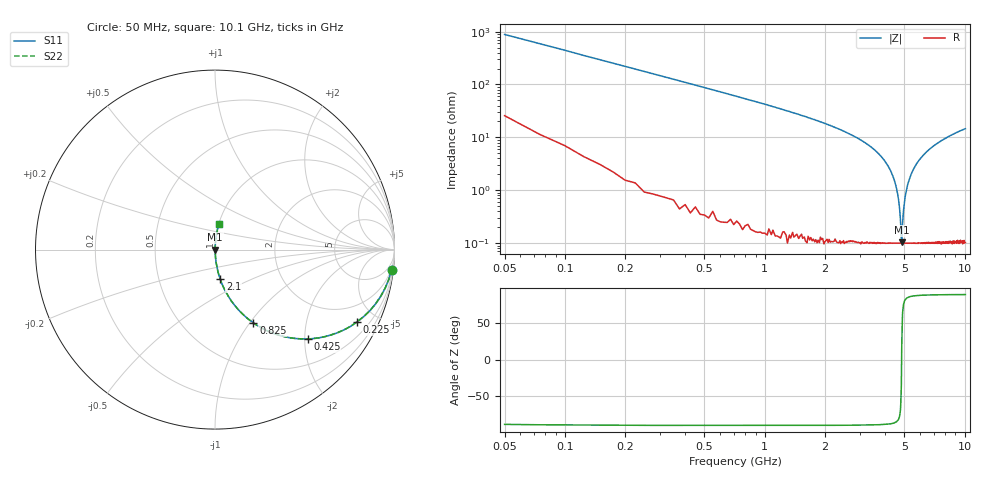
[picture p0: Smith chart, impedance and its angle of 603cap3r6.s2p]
! AVX Thin Film Operation		Date: November 2004
! Description: Accu-P® Series, Thin Film, SMD, RF Capacitor
! Part Number: 06035J3R6ABT
! 50 MHz  -  10.05 GHz
! Serial Measurements
# hz S db R 50
!	S11		S21		S12		S22
!	dB	Phase	dB	Phase	dB	Phase	dB	Phase
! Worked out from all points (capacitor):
!   400 points, 50 MHz to 10.1 GHz, reference 50 ohm
!   read as one part in series: C = 3.6 pF near 100 MHz
!   lowest |Z| = 104 mohm at 4.85 GHz (marker M1)
!   series resonance near 4.844 GHz, so ESL is about 300 pH
!   S11 on the Smith chart (normalised r, x): 50 MHz: 2, -18; 225 MHz: 1.03, -3.93; 425 MHz: 1.01, -2.06; 825 MHz: 1.00, -1.04; 2.1 GHz: 1.00, -0.34; 10.1 GHz: 1.00, +0.29
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5e7  -0.08 -6.4  -19.00 81.9  -19.00 81.9  -0.08 -6.4
1.25e8  -0.36 -15.7  -11.30 73.6  -11.30 73.6  -0.36 -15.7
2.25e8  -1.03 -26.9  -6.88 62.7  -6.88 62.7  -1.03 -26.9
4.25e8  -2.89 -44.0  -3.17 45.8  -3.17 45.8  -2.89 -44.0
8.25e8  -6.73 -62.3  -1.05 27.4  -1.05 27.4  -6.73 -62.3
1.73e9  -13.20 -77.1  -0.22 12.6  -0.22 12.6  -13.20 -77.1
2.1e9  -15.50 -79.9  -0.13 9.7  -0.13 9.7  -15.50 -79.9
3.4e9  -23.60 -85.3  -0.03 3.8  -0.03 3.8  -23.60 -85.3
4.13e9  -30.60 -86.4  -0.01 1.7  -0.01 1.7  -30.60 -86.4
4.48e9  -36.80 -85.2  -0.01 0.8  -0.01 0.8  -36.80 -85.2
4.63e9  -41.50 -82.7  -0.01 0.5  -0.01 0.5  -41.50 -82.7
4.73e9  -46.70 -77.2  -0.01 0.3  -0.01 0.3  -46.70 -77.2
4.85e9  -59.70 14.9  -0.01 -0.0  -0.01 -0.0  -59.70 14.9
4.9e9  -52.50 64.8  -0.01 -0.1  -0.01 -0.1  -52.50 64.8
4.95e9  -47.70 75.7  -0.01 -0.2  -0.01 -0.2  -47.70 75.7
5.08e9  -41.30 82.8  -0.01 -0.5  -0.01 -0.5  -41.30 82.8
5.25e9  -36.60 85.3  -0.01 -0.8  -0.01 -0.8  -36.60 85.3
5.6e9  -31.50 86.3  -0.01 -1.5  -0.01 -1.5  -31.50 86.3
6.1e9  -27.40 86.2  -0.02 -2.4  -0.02 -2.4  -27.40 86.2
6.75e9  -24.20 85.5  -0.03 -3.5  -0.03 -3.5  -24.20 85.5
8.43e9  -19.50 83.4  -0.06 -6.1  -0.06 -6.1  -19.50 83.4
1.01e10  -16.80 81.3  -0.10 -8.3  -0.10 -8.3  -16.80 81.3
